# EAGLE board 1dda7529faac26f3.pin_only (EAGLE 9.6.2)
REV: C

Size 25.4 x 17.78 mm. Coordinates in mm from the lower left corner, seen from the top.
Outline: 0,15.24 0,2.54 arc90 2.54,0 22.86,0 arc90 25.4,2.54 25.4,15.24 arc90 22.86,17.78 2.54,17.78 arc90 0,15.24
Copper layers (1*16): Top 0.035mm / dielectric 1.5mm / Bottom 0.035mm
Design rules "adafruit *": minimum track width 8mil, minimum drill 15.5mil, track to track 8mil, track to pad 8mil, pad to pad 8mil, via to via 8mil, smd to smd 8mil, copper to edge 10mil, drill to drill 8mil, minimum pad ring 10mil, minimum via ring 8mil, stop-mask expansion 2mil, vias tented up to drill 20mil, thermal gap 10mil
Net classes: 1 highpower: width 0.305 mm, drill 0.483 mm; 2 lowpower: width 0.254 mm, drill 0.483 mm

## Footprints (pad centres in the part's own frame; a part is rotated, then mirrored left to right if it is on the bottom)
0603-NO = smd 1.075 x 1: 1 -0.85,0; 2 0.85,0
_0805MP = smd 1.2 x 1.3: 1 -1.016,0; 2 1.016,0
0805-NO = smd 1.24 x 1.5: 1 -0.95,0; 2 0.95,0
JST_SH4 = smd 0.6 x 1.55: 1 -1.5,2.514; 2 -0.5,2.514; 3 0.5,2.514; 4 1.5,2.514 | smd 1.2 x 1.8: MT1 -2.8,-1.386; MT2 2.8,-1.386
CHIPLED_0603_NOOUTLINE = smd 0.8 x 0.8: A 0,-0.75; C 0,0.75
SOD-323 = smd 1.35 x 0.8: A 1.27,0; C -1.27,0
FIDUCIAL_1MM = smd 1 x 1: 1 0,0
1X06_ROUND_70 = drill 1 pad 1.778: 1 -6.35,0; 2 -3.81,0; 3 -1.27,0; 4 1.27,0; 5 3.81,0; 6 6.35,0
1X04_ROUND = drill 1 pad 1.778: 1 -3.81,0; 2 -1.27,0; 3 1.27,0; 4 3.81,0
SOT363 = smd 0.5 x 0.5: 1 -0.75,-0.9; 3 0.75,-0.9; 4 0.75,0.9; 6 -0.75,0.9 | smd 0.4 x 0.5: 2 0,-0.9; 5 0,0.9
RESPACK_4X0603 = smd 0.45 x 0.9: 1 -1.3,-0.85; 2 -0.4,-0.85; 3 0.4,-0.85; 4 1.3,-0.85; 5 1.3,0.85; 6 0.4,0.85; 7 -0.4,0.85; 8 -1.3,0.85
SOLDERJUMPER_CLOSEDWIRE = smd 1.168 x 1.6: 1 -0.762,0; 2 0.762,0 | smd 0.635 x 0.203: WIRE 0,0
LGA14 = smd 0.5 x 1.2: 1 2,1.1; 2 1.2,1.1; 3 0.4,1.1; 4 -0.4,1.1; 5 -1.2,1.1; 6 -2,1.1; 8 -2,-1.1; 9 -1.2,-1.1; 10 -0.4,-1.1; 11 0.4,-1.1; 12 1.2,-1.1; 13 2,-1.1 | smd 1.2 x 0.5: 7 -2.1,0; 14 2.1,0
SOT23-5 = smd 0.55 x 1.2: 1 -0.95,-1.3; 2 0,-1.3; 3 0.95,-1.3; 4 0.95,1.3; 5 -0.95,1.3
MOUNTINGHOLE_2.5_PLATED = drill 2.5 pad 3.2: P$1 0,0

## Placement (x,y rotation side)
C1  0.1uF  [0603-NO]  12.95,11.18 0 top
C2  10uF  [_0805MP]  7.37,5.52 0 top
C3  10uF  [0805-NO]  5.84,12.57 90 top
CONN3  STEMMA_I2C_QT  [JST_SH4]  22.73,8.89 90 top
CONN4  STEMMA_I2C_QT  [JST_SH4]  2.67,8.89 270 top
D1  GREEN  [CHIPLED_0603_NOOUTLINE]  3.56,12.57 90 top
D2  1N4148  [SOD-323]  19.68,12.7 0 top
FID3  FIDUCIAL_1MM  [FIDUCIAL_1MM]  20.26,0.83 0 top
FID4  FIDUCIAL_1MM  [FIDUCIAL_1MM]  1.97,8.89 0 top
JP1  [1X06_ROUND_70]  12.7,2.54 0 top
JP2  [1X04_ROUND]  12.7,15.24 0 top
Q2  BSS138  [SOT363]  17.78,6.1 90 top
R1  10K  [RESPACK_4X0603]  8.64,12.06 0 top
R3  10K  [RESPACK_4X0603]  17.72,9.72 270 top
SJ1  [SOLDERJUMPER_CLOSEDWIRE]  6.6,12.7 180 bottom
U1  ADXL343  [LGA14]  12.7,8.64 0 top
U2  AP2112K-3.3  [SOT23-5]  7.75,8.51 0 top
U$1  MOUNTINGHOLE2.5  [MOUNTINGHOLE_2.5_PLATED]  2.54,15.24 0 top
U$4  [ADAFRUIT_3.5MM]  4.32,14.1 0 top
U$11  [ADAFRUIT_3.5MM]  21.27,14.16 0 bottom
U$17  MOUNTINGHOLE2.5  [MOUNTINGHOLE_2.5_PLATED]  22.86,15.24 0 top
U$19  MOUNTINGHOLE2.5  [MOUNTINGHOLE_2.5_PLATED]  2.54,2.54 0 top
U$21  MOUNTINGHOLE2.5  [MOUNTINGHOLE_2.5_PLATED]  22.86,2.54 0 top
U$25  [PCBFEAT-REV-040]  3.75,6.29 0 bottom
U$30  [STEMMAQT]  22.48,4.45 90 bottom
U$31  [STEMMAQT]  2.92,13.34 270 bottom

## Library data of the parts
C1-C3 CONN3 CONN4 D1 D2 JP1 JP2 Q2 R1 R3 SJ1 U1 U$4 U$11 U$25 = microbuilder
FID3 FID4 = microbuilder; BOM: EXCLUDE
U2 = adafruit_power
U$1 U$17 U$19 U$21 = adafruit_electromech; BOM: EXCLUDE
U$30 U$31 = silks

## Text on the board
tPlace: GND | I2 | SDO | CS | Z | Y | X | ADXL345 | on | 3Vo | SCL | INT | VIN | GND | SDA
bPlace: I2C addr 0x53 | LED | Analog Devices Inc. / ADXL345 Digital MEMS / Accelerometer / ±2g ±4g ±8g ±16g | VLogic/Vcc: 3-5VDC

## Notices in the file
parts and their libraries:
microbuilder: This work is placed in the public domain, and may be freely used for commercial and non-commercial work with the following conditions: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
